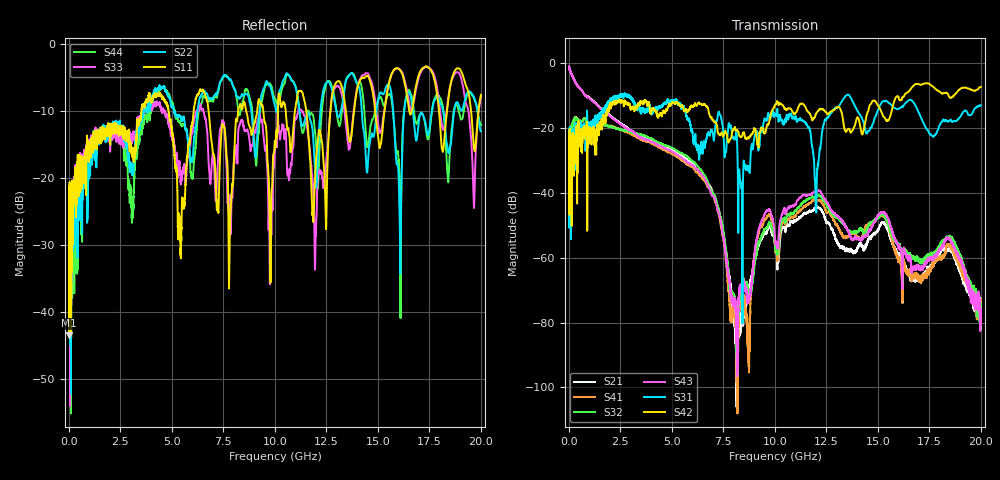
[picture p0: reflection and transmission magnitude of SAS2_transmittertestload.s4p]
! SAS 2.0 test load s-parameter file, representing performance of the
! Molex miniSAS 10-meter cable assembly.
! Model includes test fixture effects, comprised of trace loss (55 mm of
! 7-mil single-ended stripline trace in 4000-13 PC board material) and
! connector SMT attach.
! Frequency range of coverage is 10 MHz to 20 GHz, in 1 MHz steps.
! Model Node Map:
! Input port (pin)	Output port (pin)
! 1 (B5)		2 (A5)
! 3 (B6)		4 (A6)
# MHz S MA R 50.00
! FREQ  S11  S12  S13  S14
!  S21  S22  S23  S24
!  S31  S32  S33  S34
!  S41  S42  S43  S44
!  MAG  ANG  MAG  ANG  MAG  ANG  MAG  ANG
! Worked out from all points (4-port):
!   19991 points, 10 MHz to 20 GHz, reference 50 ohm
!   strongest paths, dB at 10 MHz, 5.007 GHz, 10.01 GHz, 15 GHz, 20 GHz:
!     S42: -27.1, -12.0, -12.9, -13.1, -7.4
!     S31: -27.4, -11.3, -16.0, -14.5, -13.1
!     S43: -1.0, -27.3, -54.2, -46.9, -76.6
!     S32: -33.1, -26.1, -56.1, -47.7, -75.2
!     S41: -33.8, -28.1, -56.6, -47.4, -76.1
!     S21: -1.1, -26.6, -56.0, -51.4, -73.9
!   lowest |S11| = -43.5 dB at 12 MHz (marker M1), VSWR 1.01, Z = 50.4 - j0.509 ohm
!   |S11| at or under -10 dB: start of sweep to 3.518 GHz; 4.839 GHz to 6.052 GHz (1.212 GHz wide, 22.3 % of centre); 6.783 GHz to 8.216 GHz (1.434 GHz wide, 19.1 % of centre)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
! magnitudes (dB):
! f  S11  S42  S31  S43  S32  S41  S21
! 10 MHz  -26.1  -27.1  -27.4  -1.0  -33.1  -33.8  -1.1
! 12 MHz  -43.5  -46.7  -50.8  -1.0  -27.1  -27.1  -1.0
! 6.095 GHz  -9.1  -12.7  -22.9  -31.9  -30.6  -32.8  -31.6
! 8.142 GHz  -11.3  -20.8  -21.8  -82.9  -86.0  -85.8  -100.9
! 9.555 GHz  -12.0  -21.0  -17.3  -45.9  -51.1  -48.0  -52.6
! 12.12 GHz  -13.1  -14.6  -30.3  -39.4  -40.8  -42.3  -44.6
! 20 GHz  -7.5  -7.4  -13.1  -76.6  -75.2  -76.1  -73.9
